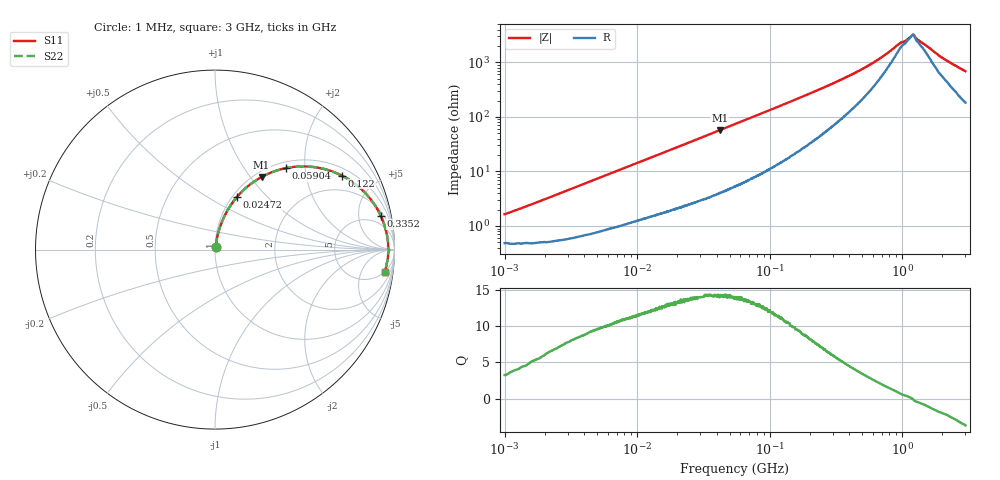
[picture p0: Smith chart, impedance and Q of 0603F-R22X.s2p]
!s-Parameter Generated by FASTRON Sdn. Bhd.
!FASTRON P/N : 0603F-R22X
!Keysight Technologies: E4991B_MY54100416_A.01.15
!Date: Wed Jun 19 15:28:58 2024
!Version  :Rev00  Wed Jun 19 15:28:58 2024
!Data & Calibration Information:
!Freq  S11  S21  S12  S22
!PortZ  Port1:50+j0  Port2:50+j0
!When reading reference impedance value at option line is always used.
! Remarks : This data is being provided solely for informational purposes.
# Hz S dB R 50
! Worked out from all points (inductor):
!   1601 points, 1 MHz to 3 GHz, reference 50 ohm
!   read as one part in series: L = 246 nH near 1.041 MHz
!   highest Q = 14.3 at 42.01 MHz (marker M1), where L = 215 nH
!   self-resonance near 1.196 GHz
!   S11 on the Smith chart (normalised r, x): 1 MHz: 1.01, +0.03; 24.72 MHz: 1.05, +0.68; 59.04 MHz: 1.12, +1.58; 122 MHz: 1.29, +3.23; 335.2 MHz: 2.70, +9.14; 3 GHz: 5, -13
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1000000  -35.70 72.0  -0.04 -0.9  -0.04 -0.9  -35.70 72.0
3804036  -25.00 80.2  -0.07 -3.2  -0.07 -3.2  -25.00 80.2
7898269  -19.00 78.3  -0.14 -6.4  -0.14 -6.4  -19.00 78.3
1.447069e7  -14.10 74.1  -0.31 -11.3  -0.31 -11.3  -14.10 74.1
2.471848e7  -10.00 67.5  -0.67 -18.3  -0.67 -18.3  -10.00 67.5
3.271304e7  -8.01 62.6  -1.01 -23.4  -1.01 -23.4  -8.01 62.6
4.201274e7  -6.36 57.3  -1.48 -28.6  -1.48 -28.6  -6.36 57.3
5.504702e7  -4.79 50.8  -2.19 -35.1  -2.19 -35.1  -4.79 50.8
5.904167e7  -4.42 49.0  -2.42 -36.8  -2.42 -36.8  -4.42 49.0
8.422788e7  -2.86 39.7  -3.87 -45.9  -3.87 -45.9  -2.86 39.7
1.219755e8  -1.74 30.2  -5.94 -54.6  -5.94 -54.6  -1.74 30.2
1.582265e8  -1.22 24.2  -7.69 -59.8  -7.69 -59.8  -1.22 24.2
2.083556e8  -0.85 18.8  -9.77 -64.1  -9.77 -64.1  -0.85 18.8
3.351655e8  -0.51 11.5  -13.90 -68.0  -13.90 -68.0  -0.51 11.5
5.391547e8  -0.36 6.3  -18.80 -65.8  -18.80 -65.8  -0.36 6.3
7.925923e8  -0.32 3.0  -24.10 -53.4  -24.10 -53.4  -0.32 3.0
9.633956e8  -0.31 1.5  -27.30 -35.2  -27.30 -35.2  -0.31 1.5
1.070143e9  -0.31 0.8  -28.40 -21.9  -28.40 -21.9  -0.31 0.8
1.176881e9  -0.28 0.2  -30.00 -5.2  -30.00 -5.2  -0.28 0.2
1.212752e9  -0.26 -0.2  -30.50 5.6  -30.50 5.6  -0.26 -0.2
1.970482e9  -0.34 -3.9  -22.30 58.4  -22.30 58.4  -0.34 -3.9
3e9  -0.40 -7.6  -17.20 67.1  -17.20 67.1  -0.40 -7.6
